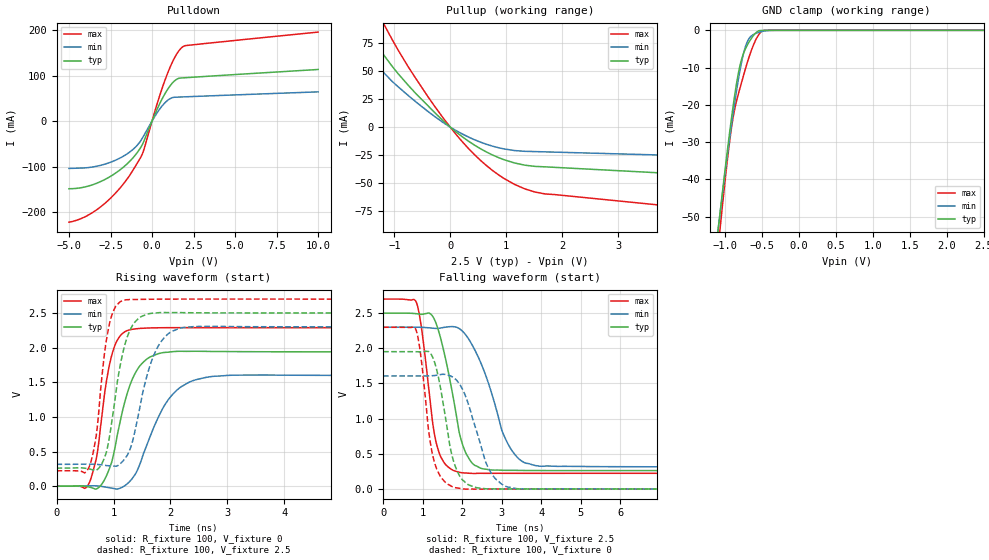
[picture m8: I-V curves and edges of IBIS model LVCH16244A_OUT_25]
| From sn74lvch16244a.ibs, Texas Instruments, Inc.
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[Model]   LVCH16244A_OUT_25
Model_type  3-state
Enable   Active-Low
Vref =   0
Rref =   500
Cref =   30p
Vmeas =   1.25
| variable   typ   min   max
C_comp   4.83pF   4.40pF   6.01pF
| C_pullup   6.00pF   3.90pF   9.12pF
| C_pulldown   7.52pF   5.42pF   9.58pF
| C_tri-state   4.83pF   4.40pF   6.01pF
[Temperature Range]   40   100   -40
| Ambient temperature   25   85   -40
[Voltage range]   2.5   2.3   2.7
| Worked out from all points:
|   slope of the pulldown table from 0 to 0.375 V, typ, clamps not added: 11.9 ohm
|   slope of the pullup table from 0 to 0.375 V, typ, clamps not added: 26.5 ohm
|   GND clamp passes 1 mA (typ) near -0.59 V on its own axis
|   rising waveform, R_fixture 100, V_fixture 0: 20-80 % time 353ps typ, 526ps min, 240ps max; typ from 0 V to 1.94 V
|   falling waveform, R_fixture 100, V_fixture 2.5: 20-80 % time 474ps typ, 712ps min, 329ps max; typ from 2.5 V to 0.262 V
|   rising waveform, R_fixture 100, V_fixture 2.5: 20-80 % time 275ps typ, 361ps min, 201ps max; typ from 0.262 V to 2.5 V
|   falling waveform, R_fixture 100, V_fixture 0: 20-80 % time 377ps typ, 536ps min, 297ps max; typ from 1.95 V to 0 V
[GND Clamp]
| LVCH16244A_OUT_25
|   Voltage   I(typ)   I(min)   I(max)
-5V       -855.7mA   -797.6mA   -953.2mA
-1.09V    -54.36mA   -53.97mA   -59.22mA
-1.06V    -49.06mA   -49.09mA   -53.29mA
-955mV    -31.29mA   -32.66mA   -33.81mA
-900mV    -22.75mA   -24.6mA    -25.4mA
-840mV    -14.58mA   -16.51mA   -19.19mA
-790mV    -9.382mA   -10.63mA   -15.45mA
-730mV    -5.543mA   -5.229mA   -11.2mA
-675mV    -3.361mA   -2.41mA    -7.57mA
-570mV    -549.4uA   -770.8uA   -2.257mA
-490mV    -16.56uA   -280.7uA   -181.4uA
2.5V      9.148pA    37.98nA    -17.36pA
[Pulldown]
| LVCH16244A_OUT_25
|   Voltage   I(typ)   I(min)   I(max)
-5V       -148.4mA   -103.9mA   -221.8mA
-4.05V    -144.6mA   -102.7mA   -210.3mA
-3.075V   -132.4mA   -96.92mA   -187.6mA
-2.11V    -112mA     -84.37mA   -154.5mA
-1.27V    -85.53mA   -65.87mA   -114.9mA
-850mV    -67.03mA   -51.33mA   -89.83mA
-540mV    -48.37mA   -34.68mA   -68.09mA
230mV     19.76mA    13.93mA    28.68mA
750mV     58.22mA    39.1mA     86.73mA
1.33V     87.32mA    52.22mA    137mA
1.83V     94.73mA    52.98mA    162.4mA
10V       113.2mA    64.1mA     195.3mA
[Pullup]
| LVCH16244A_OUT_25
|   Voltage   I(typ)   I(min)   I(max)
-5V       107mA      39.78mA    366.9mA
-3.895V   252mA      53.48mA    373.6mA
-3.68V    242.4mA    66.07mA    353.2mA
-3.58V    236.9mA    97.7mA     343.4mA
-1.875V   115.8mA    88.65mA    164.7mA
-1.47V    84.95mA    64.9mA     120.5mA
-1.2V     65.32mA    49.39mA    93.48mA
-395mV    18.99mA    13.91mA    27.01mA
320mV     -12.34mA   -8.718mA   -18.78mA
965mV     -29.2mA    -19.52mA   -46.04mA
1.515V    -35.13mA   -21.87mA   -58.07mA
10V       -57.52mA   -33.56mA   -101.4mA
[Ramp]
| LVCH16244A_OUT_25
| variable   typ   min   max
dV/dt_r   1.19/3.66E-10   0.99/5.55E-10   1.39/2.50E-10
dV/dt_f   1.34/4.94E-10   1.20/7.58E-10   1.49/3.34E-10
R_load = 100
[Rising Waveform]
| LVCH16244A_OUT_25
R_fixture =   100
C_fixture =   0
L_fixture =   0
V_fixture =   0
V_fixture_min = 0
V_fixture_max = 0
|   Time   V(typ)   V(min)   V(max)
0s        -35.86uV   -73.74uV   -15.21uV
555ps     -8.022mV   5.638mV    18.92mV
700ps     -38.65mV   5.388mV    405.4mV
800ps     36.62mV    -3.652mV   1.04V
1.045ns   640.5mV    -39.84mV   2.072V
1.26ns    1.39V      49.31mV    2.251V
1.49ns    1.763V     380.2mV    2.278V
2.105ns   1.946V     1.381V     2.288V
3.105ns   1.942V     1.603V     2.288V
49.99ns   1.94V      1.597V     2.288V
[Falling Waveform]
| LVCH16244A_OUT_25
R_fixture =   100
C_fixture =   0
L_fixture =   0
V_fixture =   2.5
V_fixture_min = 2.3
V_fixture_max = 2.7
|   Time   V(typ)   V(min)   V(max)
0s        2.5V       2.3V       2.7V
840ps     2.492V     2.3V       2.657V
990ps     2.483V     2.298V     2.215V
1.265ns   2.447V     2.286V     903.1mV
1.535ns   1.965V     2.297V     383.2mV
2.02ns    617.6mV    2.237V     229mV
2.33ns    333.1mV    1.968V     221.1mV
3.195ns   265.1mV    607.1mV    222.6mV
3.97ns    262.1mV    323.8mV    222.6mV
49.99ns   261.9mV    316.3mV    222.8mV
[Rising Waveform]
| LVCH16244A_OUT_25
R_fixture =   100
C_fixture =   0
L_fixture =   0
V_fixture =   2.5
V_fixture_min = 2.3
V_fixture_max = 2.7
|   Time   V(typ)   V(min)   V(max)
0s        261.9mV    316.2mV    222.8mV
565ps     250.6mV    318.9mV    265.5mV
700ps     231.4mV    316.1mV    747.4mV
790ps     316.7mV    308.4mV    1.526V
970ps     932.4mV    293mV      2.467V
1.12ns    1.753V     325.6mV    2.662V
1.275ns   2.226V     504.9mV    2.693V
1.77ns    2.502V     2V         2.699V
2.42ns    2.502V     2.304V     2.7V
49.99ns   2.5V       2.3V       2.7V
[Falling Waveform]
| LVCH16244A_OUT_25
R_fixture =   100
C_fixture =   0
L_fixture =   0
V_fixture =   0
V_fixture_min = 0
V_fixture_max = 0
|   Time   V(typ)   V(min)   V(max)
0s        1.952V     1.607V     2.299V
830ps     1.951V     1.607V     2.267V
955ps     1.95V      1.607V     1.889V
1.22ns    1.911V     1.61V      578.9mV
1.41ns    1.563V     1.623V     220.5mV
1.755ns   454.5mV    1.593V     32.78mV
2.05ns    110.5mV    1.371V     -563.9uV
2.715ns   1.073mV    246.1mV    -232.1uV
3.445ns   392.5uV    1.264mV    -51.09uV
49.99ns   -8.822uV   -1.313uV   -3.331uV
